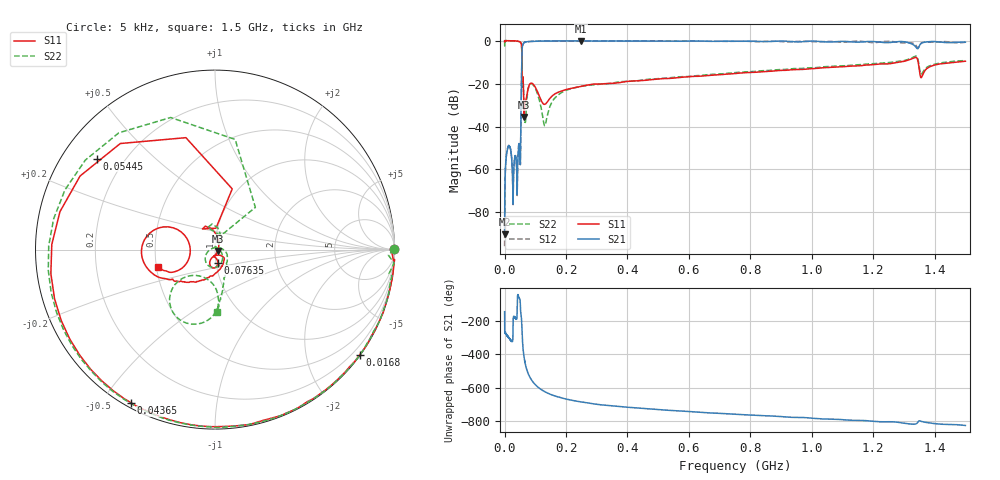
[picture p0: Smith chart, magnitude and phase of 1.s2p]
#  HZ  S  MA  R  50.00
! Rohde & Schwarz Vector Network Analyzer
! Rohde-Schwarz,ZNL6-2Port,1323001206101378,1.50.1.34-21.10.1.104
! Created: UTC 7/25/2024, 5:52:27 AM
! freq[Hz]  mag:S11  ang:S11  mag:S21  ang:S21  mag:S12  ang:S12  mag:S22  ang:S22
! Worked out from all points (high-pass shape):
!   10001 points, 5 kHz to 1.5 GHz, reference 50 ohm
!   highest |S21| = -0.08 dB at 247.4 MHz (marker M1); lowest = -90.1 dB at 5 kHz (marker M2)
!   |S21| within 3 dB of the highest: 57.58 MHz to 1.339 GHz (1.282 GHz wide, 184 % of centre); 1.348 GHz to end of sweep
!   lowest |S11| = -35.5 dB at 63.75 MHz (marker M3), VSWR 1.03, Z = 51.5 - j0.788 ohm
!   |S11| at or under -10 dB: 56.8 MHz to 1.285 GHz (1.228 GHz wide, 183 % of centre); 1.346 GHz to 1.469 GHz (123 MHz wide, 8.74 % of centre)
!   |S22| runs from -39.6 to 0.1 dB; largest |S21 - S12| = 0.11
!   S11 on the Smith chart (normalised r, x): 5 kHz: open; 16.8 MHz: 0.02, -3.07; 43.65 MHz: 0.02, -0.59; 54.45 MHz: 0.10, +0.34; 76.35 MHz: 1.02, -0.15; 1.5 GHz: 0.51, -0.11
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5000  1 0.1  3.111e-05 -144.1  1.637e-05 152.4  0.9984 0.1
8704971  0.9975 -17.8  0.002889 72.7  0.002941 68.2  0.9979 -19.8
1.680494e7  0.9971 -36.1  0.003432 52.1  0.003419 51.4  0.9973 -40.3
3.285489e7  0.9898 -77.9  0.001868 -176.8  0.001863 -177.1  0.9901 -87.1
4.365485e7  0.9741 -118.6  0.002236 -44.6  0.002217 -49.6  0.9704 -133.0
4.710484e7  0.9588 -138.3  0.004019 -60.4  0.004045 -58.4  0.9523 -154.0
5.445482e7  0.8304 142.4  0.07513 -173.7  0.0748 -174.7  0.8156 119.8
6.375479e7  0.01682 -27.1  0.8994 -63.3  0.8993 -63.0  0.02106 64.2
6.900477e7  0.04035 -94.6  0.9327 -111.9  0.9326 -111.7  0.01618 29.0
7.635475e7  0.07645 -77.6  0.9517 -154.2  0.9515 -154.1  0.07186 -55.5
9.645468e7  0.09015 -108.0  0.9706 144.1  0.9703 144.4  0.08607 -126.4
1.216546e8  0.03723 -98.4  0.9805 104.7  0.9818 104.9  0.02132 169.7
1.321546e8  0.03327 -69.7  0.9804 93.6  0.9832 93.8  0.0108 82.2
2.473542e8  0.08592 -56.7  0.9908 33.9  0.9861 33.4  0.08571 -36.3
2.500542e8  0.08669 -57.3  0.9907 33.1  0.9861 32.5  0.08644 -36.9
5.001033e8  0.1289 -86.6  0.9829 -12.4  0.9855 -11.3  0.13 -63.4
7.500025e8  0.1719 -107.5  0.9696 -41.0  0.9688 -38.9  0.1807 -73.7
1.000052e9  0.2229 -126.7  0.9807 -64.2  0.946 -63.0  0.2344 -79.9
1.250101e9  0.2893 -145.3  0.9032 -85.8  0.9704 -86.0  0.3084 -86.0
1.336951e9  0.409 -174.6  0.7367 -100.0  0.809 -99.4  0.4369 -108.7
1.35855e9  0.1468 -164.9  0.8867 -84.8  0.8957 -86.1  0.1725 -102.6
1.5e9  0.3331 -162.8  0.9228 -108.1  0.9201 -104.9  0.3483 -88.1
